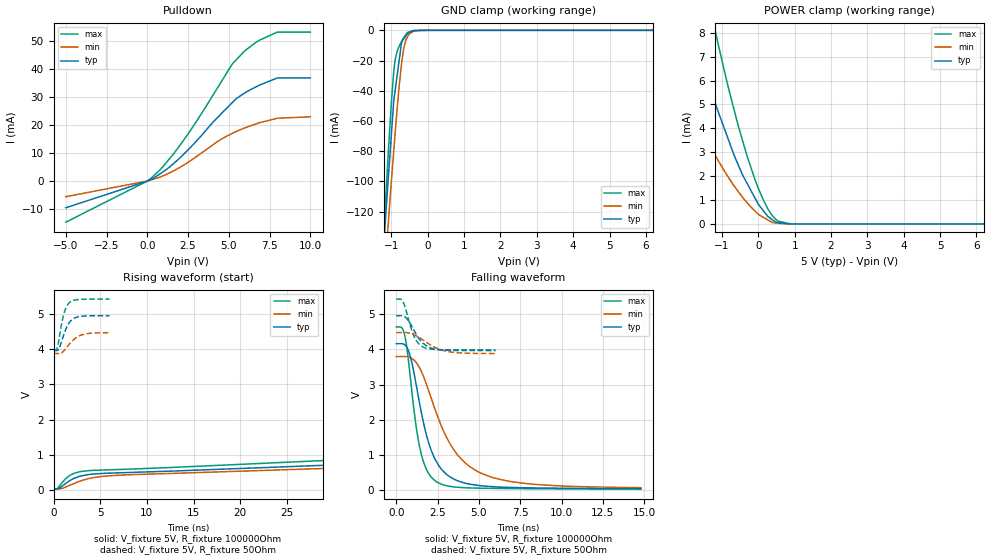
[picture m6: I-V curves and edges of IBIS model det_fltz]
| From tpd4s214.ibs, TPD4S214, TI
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|   det_fltz Model
[Model]   det_fltz
Model_type   Open_drain
Polarity   Inverting
Vmeas = 2.5
Vref = 5
Cref = 2pF
Rref = 100000
|   typ   min   max
|   (nom PVT)   (fast PVT)   (slow PVT)
C_comp   1.813e-12   1.693e-12   1.935e-12
| Where nom  PVT is Nominal Process, 5V, 27C
|   Fast PVT is Strong Process,  5.5V, -40C
|   Slow PVT is Weak Process,   4.5V, 125C
[Voltage Range]   5   4.5   5.5
|Junction Temperature
[Temperature Range]   27   125   -40
[Pullup Reference]   5   4.5   5.5
[Pulldown Reference]   0   0   0
[Power Clamp Reference]   5   4.5   5.5
[GND Clamp Reference]   0   0   0
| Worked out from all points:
|   slope of the pulldown table from 0 to 0.75 V, typ, clamps not added: 308 ohm
|   GND clamp passes 1 mA (typ) near -0.48 V on its own axis
|   POWER clamp passes 1 mA (typ) near -0.06 V on its own axis
|   falling waveform, V_fixture 5V, R_fixture 100000Ohm: 20-80 % time 1.29ns typ, 2.29ns min, 826ps max; typ from 4.17 V to 0.032 V
|   rising waveform, V_fixture 5V, R_fixture 100000Ohm: 20-80 % time 344ns typ, 366ns min, 323ns max; typ from 0.019 V to 4.17 V
|   falling waveform, V_fixture 5V, R_fixture 50Ohm: 20-80 % time 835ps typ, 1.31ns min, 611ps max; typ from 4.96 V to 3.97 V
|   rising waveform, V_fixture 5V, R_fixture 50Ohm: 20-80 % time 896ps typ, 1.33ns min, 690ps max; typ from 3.97 V to 4.96 V
[Pulldown]
|   Voltage   I(typ)   I(min)   I(max)
-5V       -9.53mA    -5.578mA   -14.66mA
0V        0A         0A         0A
775.5mV   2.536mA    1.39mA     3.973mA
1.672V    6.545mA    3.835mA    10.14mA
2.558V    11.45mA    6.865mA    17.27mA
4.253V    22.33mA    13.9mA     32.71mA
5.192V    27.85mA    16.93mA    41.54mA
5.43V     29.25mA    17.6mA     43.06mA
5.957V    31.31mA    18.89mA    46.31mA
6.886V    34.2mA     20.83mA    50.22mA
7.975V    36.75mA    22.39mA    53.1mA
10V       36.75mA    22.9mA     53.1mA
[GND Clamp]
|   Voltage   I(typ)   I(min)   I(max)
-5V       -1.684A    -1.564A    -1.883A
-1.21V    -142.5mA   -168.5mA   -134mA
-1.183V   -132.7mA   -159.5mA   -122.8mA
-1.083V   -97.44mA   -126.9mA   -80.33mA
-995.5mV  -67.34mA   -98.53mA   -46.31mA
-935mV    -46.64mA   -79.89mA   -27.47mA
-891mV    -38.75mA   -66.33mA   -18.82mA
-720mV    -8.068mA   -21.95mA   -7.286mA
-670.5mV  -5.889mA   -13.37mA   -5.291mA
-598.5mV  -3.581mA   -6.108mA   -2.701mA
-435mV    -294.4uA   -1.273mA   -493.2uA
10V       0A         0A         0A
[POWER Clamp]
|   Voltage   I(typ)   I(min)   I(max)
-5V       84.53mA    37.68mA    167.4mA
-2.695V   13.33mA    8.001mA    28.32mA
-2.42V    11.66mA    6.995mA    17.71mA
-1.375V   5.953mA    3.413mA    9.414mA
-1.14V    4.848mA    2.757mA    7.776mA
-808.5mV  3.466mA    1.919mA    5.611mA
-302.5mV  1.68mA     879.5uA    2.807mA
27.5mV    769.7uA    371.1uA    1.386mA
396mV     165.1uA    54.04uA    323.7uA
528mV     60.2uA     33.15uA    123.4uA
880mV     610.4nA    758.5nA    1.076uA
10V       0A         0A         0A
[Ramp]
R_load = 100000
|   typ   min   max
dV/dt_r   2.56528/3.43037e-07   2.2967/3.65903e-07   2.83444/3.23219e-07
dV/dt_f   2.56528/1.30475e-09   2.29673/2.34181e-09   2.83444/8.27065e-10
[Falling Waveform]
V_fixture = 5V
V_fixture_min = 4.5V
V_fixture_max = 5.5V
R_fixture = 100000Ohm
|   Time   V(typ)   V(min)   V(max)
0s        4.166V     3.797V     4.642V
500ps     4.14V      3.799V     4.428V
900ps     3.705V     3.755V     2.972V
1.2ns     2.996V     3.629V     1.794V
1.5ns     2.233V     3.388V     1.033V
1.9ns     1.428V     2.9V       508.5mV
2.4ns     821.7mV    2.218V     238.4mV
3.7ns     258.4mV    998.3mV    73.26mV
5.6ns     97.15mV    385.3mV    42.55mV
14.8ns    32.02mV    60.16mV    17.77mV
[Rising Waveform]
V_fixture = 5V
V_fixture_min = 4.5V
V_fixture_max = 5.5V
R_fixture = 100000Ohm
|   Time   V(typ)   V(min)   V(max)
0s        19.15mV    25.43mV    13.82mV
2ns       296.8mV    153.4mV    442mV
4.2ns     444.3mV    340mV      549.3mV
158.7ns   1.905V     1.649V     2.242V
279.5ns   2.76V      2.405V     3.215V
422.5ns   3.494V     3.072V     4.028V
528ns     3.878V     3.428V     4.441V
604.6ns   4.073V     3.62V      4.613V
720ns     4.163V     3.768V     4.642V
999.9ns   4.166V     3.797V     4.642V
[Falling Waveform]
V_fixture = 5V
V_fixture_min = 4.5V
V_fixture_max = 5.5V
R_fixture = 50Ohm
|   Time   V(typ)   V(min)   V(max)
0s        4.963V     4.481V     5.437V
262ps     4.964V     4.481V     5.436V
389ps     4.961V     4.482V     5.376V
667ps     4.861V     4.478V     4.979V
1.064ns   4.548V     4.422V     4.388V
1.306ns   4.356V     4.363V     4.19V
1.602ns   4.185V     4.274V     4.071V
2.145ns   4.035V     4.107V     4.006V
3.044ns   3.979V     3.948V     3.992V
5.999ns   3.97V      3.884V     3.989V
[Rising Waveform]
V_fixture = 5V
V_fixture_min = 4.5V
V_fixture_max = 5.5V
R_fixture = 50Ohm
|   Time   V(typ)   V(min)   V(max)
0s        3.97V      3.883V     3.989V
389ps     3.968V     3.882V     4.029V
619ps     4.039V     3.88V      4.341V
877ps     4.239V     3.903V     4.74V
1.096ns   4.419V     3.957V     5.001V
1.378ns   4.615V     4.047V     5.214V
1.706ns   4.771V     4.154V     5.337V
2.312ns   4.902V     4.314V     5.411V
3.152ns   4.948V     4.425V     5.43V
5.999ns   4.962V     4.478V     5.436V
